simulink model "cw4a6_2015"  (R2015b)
settings: Solver=FixedStepAuto  SolverMode=SingleTasking  StartTime=0.0  StopTime=100  FixedStep=0.01  RelTol=1e-3
libraries: neural x31

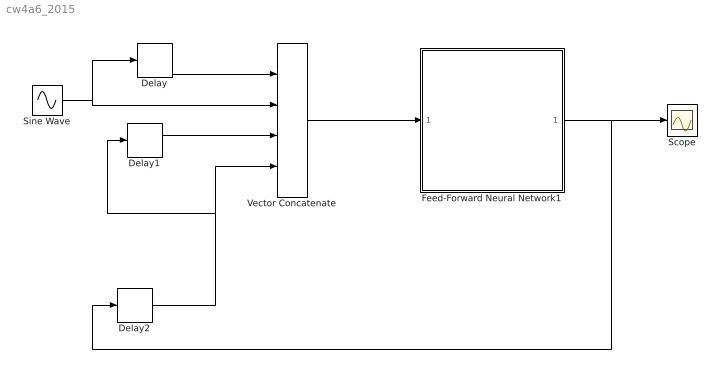
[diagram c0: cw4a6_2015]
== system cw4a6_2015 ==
  Delay : Delay  DelayLength=1  InitialCondition=0
  Delay1 : Delay  DelayLength=1  InitialCondition=0
  Delay2 : Delay  DelayLength=1  InitialCondition=0
  Feed-Forward Neural Network1 : Subsystem
  Scope : Scope
  Sine Wave : Sin  Amplitude=3  SampleTime=0
  Vector Concatenate : Concatenate  NumInputs=4
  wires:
  Vector Concatenate/1 -> Feed-Forward Neural Network1/1(Input)
  Sine Wave/1 -> Delay/1, Vector Concatenate/2
  Delay/1 -> Vector Concatenate/1
  Feed-Forward Neural Network1/1(Output) -> Scope/1, Delay2/1
  Delay1/1 -> Vector Concatenate/3
  Delay2/1 -> Delay1/1, Vector Concatenate/4

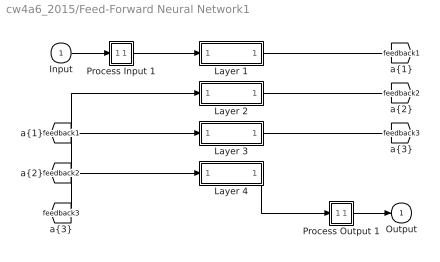
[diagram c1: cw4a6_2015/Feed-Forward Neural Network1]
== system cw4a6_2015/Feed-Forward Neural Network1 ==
  Input : Inport  PortDimensions=4  SampleTime=0.01
  Layer 1 : Subsystem
  Layer 2 : Subsystem
  Layer 3 : Subsystem
  Layer 4 : Subsystem
  Process Input 1 : Subsystem
  Process Output 1 : Subsystem
  Output : Outport  InitialOutput=0
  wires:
  Input/1 -> Process Input 1/1(x)
  Process Output 1/1(y) -> Output/1
  Process Input 1/1(p) -> Layer 1/1("p{1}")
  Layer 1/1("a{1}") -> [feedback1]
  [feedback1] -> Layer 2/1("a{1} ")
  Layer 2/1("a{2}") -> [feedback2]
  [feedback2] -> Layer 3/1("a{2} ")
  Layer 3/1("a{3}") -> [feedback3]
  [feedback3] -> Layer 4/1("a{3} ")
  Layer 4/1("a{4}") -> Process Output 1/1(a)

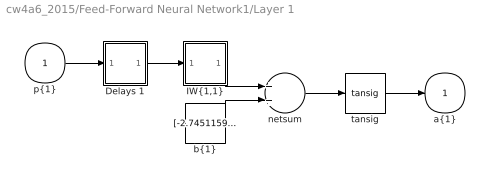
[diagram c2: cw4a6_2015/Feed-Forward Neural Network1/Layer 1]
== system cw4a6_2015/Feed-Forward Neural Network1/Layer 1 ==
  "p{1}" : Inport  PortDimensions=4  SampleTime=0.01
  Delays 1 : Subsystem
  "IW{1,1}" : Subsystem
  "b{1}" : Constant  Value=[-2.7451159693212377;-0.51927762787376885;1.1959405771862848;1.954048280311202]
  netsum : Sum  Inputs=2
  tansig : neural/Transfer Functions/tansig
  "a{1}" : Outport  InitialOutput=[0;0;0;0]
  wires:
  "p{1}"/1 -> Delays 1/1("p{1}")
  Delays 1/1("pd{1,1}") -> "IW{1,1}"/1("pd{1,1}")
  "IW{1,1}"/1("iz{1,1}") -> netsum/1
  "b{1}"/1 -> netsum/2
  netsum/1 -> tansig/1
  tansig/1 -> "a{1}"/1

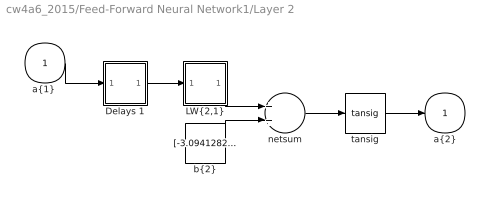
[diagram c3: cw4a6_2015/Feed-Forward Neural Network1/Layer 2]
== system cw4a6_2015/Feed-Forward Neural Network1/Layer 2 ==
  "a{1} " : Inport  PortDimensions=4  SampleTime=0.01
  Delays 1 : Subsystem
  "LW{2,1}" : Subsystem
  "b{2}" : Constant  Value=[-3.0941282887806971;2.5007190554093581;1.9491510266515135;-1.6091889436891094;1.4251518713600293;-1.2415776302483117;0.76744618770440332;-0.24724036630592988;0.4711224294363367;-0.70575018159961311;0.68364287193172868;-1.3894845729981458;1.1167616282660546;-2.0699518501358609;-2.3105194954019512;2.6036849767045065]
  netsum : Sum  Inputs=2
  tansig : neural/Transfer Functions/tansig
  "a{2}" : Outport  InitialOutput=[0;0;0;0;0;0;0;0;0;0;0;0;0;0;0;0]
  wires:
  "a{1} "/1 -> Delays 1/1("p{2}")
  Delays 1/1("pd{2,1}") -> "LW{2,1}"/1("ad{2,1}")
  "LW{2,1}"/1("lz{2,1}") -> netsum/1
  "b{2}"/1 -> netsum/2
  netsum/1 -> tansig/1
  tansig/1 -> "a{2}"/1

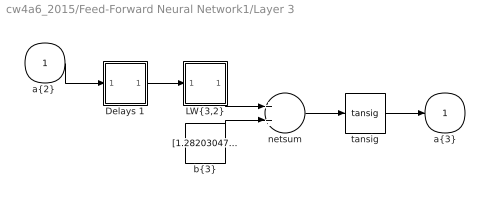
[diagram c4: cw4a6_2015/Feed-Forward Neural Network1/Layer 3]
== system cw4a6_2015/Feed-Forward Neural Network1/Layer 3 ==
  "a{2} " : Inport  PortDimensions=16  SampleTime=0.01
  Delays 1 : Subsystem
  "LW{3,2}" : Subsystem
  "b{3}" : Constant  Value=[1.2820304787533141;-0.73780855735148043;-0.35364559770692083;-1.5031025952607859]
  netsum : Sum  Inputs=2
  tansig : neural/Transfer Functions/tansig
  "a{3}" : Outport  InitialOutput=[0;0;0;0]
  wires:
  "a{2} "/1 -> Delays 1/1("p{3}")
  Delays 1/1("pd{3,2}") -> "LW{3,2}"/1("ad{3,2}")
  "LW{3,2}"/1("lz{3,2}") -> netsum/1
  "b{3}"/1 -> netsum/2
  netsum/1 -> tansig/1
  tansig/1 -> "a{3}"/1

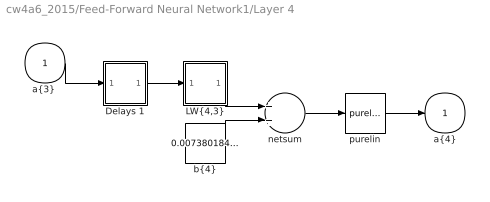
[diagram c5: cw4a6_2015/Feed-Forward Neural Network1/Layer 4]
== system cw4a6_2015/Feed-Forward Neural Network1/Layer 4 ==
  "a{3} " : Inport  PortDimensions=4  SampleTime=0.01
  Delays 1 : Subsystem
  "LW{4,3}" : Subsystem
  "b{4}" : Constant  Value=0.0073801844453347783
  netsum : Sum  Inputs=2
  purelin : neural/Transfer Functions/purelin
  "a{4}" : Outport  InitialOutput=0
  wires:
  "a{3} "/1 -> Delays 1/1("p{4}")
  Delays 1/1("pd{4,3}") -> "LW{4,3}"/1("ad{4,3}")
  "LW{4,3}"/1("lz{4,3}") -> netsum/1
  "b{4}"/1 -> netsum/2
  netsum/1 -> purelin/1
  purelin/1 -> "a{4}"/1

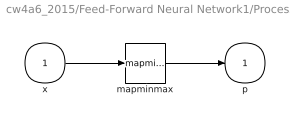
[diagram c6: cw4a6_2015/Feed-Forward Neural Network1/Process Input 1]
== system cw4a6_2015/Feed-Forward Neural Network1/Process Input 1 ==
  x : Inport  PortDimensions=4  SampleTime=0.01
  mapminmax : neural/Processing Functions/mapminmax  xmin=[-2.9999999573670899;-2.9999999573670899;-1.6037325965643041;-1.6037325965643041]  xmax=[2.9999999873508418;2.9999999873508418;1.5876018327536372;1.5876018327536372]  ymin=-1  ymax=1
  p : Outport  PortDimensions=4  SampleTime=0.01
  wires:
  x/1 -> mapminmax/1
  mapminmax/1 -> p/1

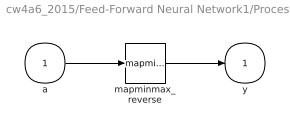
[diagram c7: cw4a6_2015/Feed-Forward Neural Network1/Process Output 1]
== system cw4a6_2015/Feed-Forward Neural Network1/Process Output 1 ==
  a : Inport  PortDimensions=1  SampleTime=0.01
  mapminmax_reverse : neural/Processing Functions/mapminmax_reverse  xmin=-1.6037325965643041  xmax=1.5876018327536372  ymin=-1  ymax=1
  y : Outport  PortDimensions=1  SampleTime=0.01
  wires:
  a/1 -> mapminmax_reverse/1
  mapminmax_reverse/1 -> y/1

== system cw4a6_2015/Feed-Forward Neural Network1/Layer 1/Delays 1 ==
  "p{1}" : Inport  PortDimensions=4  SampleTime=0.01
  mux : Mux  Inputs=1
  "pd{1,1}" : Outport
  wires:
  "p{1}"/1 -> mux/1
  mux/1 -> "pd{1,1}"/1

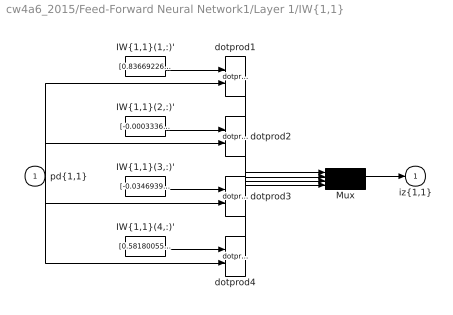
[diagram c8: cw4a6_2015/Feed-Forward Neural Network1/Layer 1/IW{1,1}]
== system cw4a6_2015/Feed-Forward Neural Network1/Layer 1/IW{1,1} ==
  "pd{1,1}" : Inport  PortDimensions=4  SampleTime=0.01
  "IW{1,1}(1,:)'" : Constant  Value=[0.83669226565768351;-0.74873759136295048;-0.96234576370289271;0.37325137038861117]
  "IW{1,1}(2,:)'" : Constant  Value=[-0.0003336744559937728;-0.00039010697089592478;-0.30642803603807789;0.60937703466284387]
  "IW{1,1}(3,:)'" : Constant  Value=[-0.034693924814063352;0.16844250588365894;0.76279626784045285;-0.17752775686451444]
  "IW{1,1}(4,:)'" : Constant  Value=[0.5818005537766594;0.90179528476757986;-0.22477921341837884;0.12222051479645338]
  Mux : Mux
  dotprod{1..4} (4 alike) : neural/Weight Functions/dotprod
  "iz{1,1}" : Outport
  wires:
  "IW{1,1}(1,:)'"/1 -> dotprod1/1
  "pd{1,1}"/1 -> dotprod1/2, dotprod2/2, dotprod3/2, dotprod4/2
  dotprod1/1 -> Mux/1
  "IW{1,1}(2,:)'"/1 -> dotprod2/1
  dotprod2/1 -> Mux/2
  "IW{1,1}(3,:)'"/1 -> dotprod3/1
  dotprod3/1 -> Mux/3
  "IW{1,1}(4,:)'"/1 -> dotprod4/1
  dotprod4/1 -> Mux/4
  Mux/1 -> "iz{1,1}"/1

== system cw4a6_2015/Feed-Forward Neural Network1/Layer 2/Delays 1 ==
  "p{2}" : Inport  PortDimensions=4  SampleTime=0.01
  mux : Mux  Inputs=1
  "pd{2,1}" : Outport
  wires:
  "p{2}"/1 -> mux/1
  mux/1 -> "pd{2,1}"/1

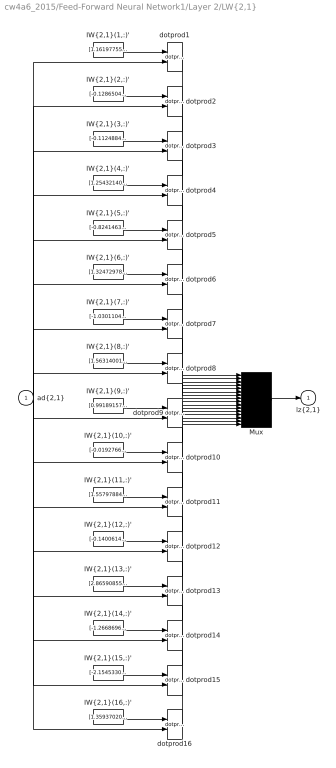
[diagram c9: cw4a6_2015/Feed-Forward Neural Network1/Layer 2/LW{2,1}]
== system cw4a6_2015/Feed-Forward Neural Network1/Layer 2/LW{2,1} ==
  "ad{2,1}" : Inport  PortDimensions=4  SampleTime=0.01
  "IW{2,1}(1,:)'" : Constant  Value=[1.1619775513977304;-2.2031284357403633;0.45459113386422795;-0.86857666926111776]
  "IW{2,1}(10,:)'" : Constant  Value=[-0.019276692855536848;0.54978083604503003;-1.3930468139942518;2.1350487871589929]
  "IW{2,1}(11,:)'" : Constant  Value=[1.5579788444873723;-1.5886105818001446;-1.0902860786850852;1.4211623229204338]
  "IW{2,1}(12,:)'" : Constant  Value=[-0.14006142548391878;-1.4133972790272766;-1.5916388419386516;1.5759542712752714]
  "IW{2,1}(13,:)'" : Constant  Value=[2.8659085537820359;0.60522502995712779;0.0058109977953483254;1.2254165100910313]
  "IW{2,1}(14,:)'" : Constant  Value=[-1.2668696691178363;2.0172300742823461;1.8445786770211106;0.26217247906200308]
  "IW{2,1}(15,:)'" : Constant  Value=[-2.1545330363134259;-0.64742657934957937;1.0991901026838413;-1.1935631889128151]
  "IW{2,1}(16,:)'" : Constant  Value=[1.3593702063748641;0.46413197701403974;2.3128596993208599;-0.12255806313010746]
  "IW{2,1}(2,:)'" : Constant  Value=[-0.12865042340396424;1.8582424739004237;1.2150803047094694;-1.2142721671715175]
  "IW{2,1}(3,:)'" : Constant  Value=[-0.11248842580797785;0.89804609193892571;1.8927709477903503;-1.8989976446848842]
  "IW{2,1}(4,:)'" : Constant  Value=[1.2543214069614295;-1.1815005524957249;-1.5671094633574423;1.5819257759203105]
  "IW{2,1}(5,:)'" : Constant  Value=[-0.82414639837216042;-1.9068075047638195;-1.8175012039809864;0.78505691762512242]
  "IW{2,1}(6,:)'" : Constant  Value=[1.3247297822434136;-1.4039801264342664;0.23930805038668623;-1.8575388549116805]
  "IW{2,1}(7,:)'" : Constant  Value=[-1.0301104085961448;-2.1013505254009393;-1.4127876628063598;0.9588134099123895]
  "IW{2,1}(8,:)'" : Constant  Value=[1.5631400167839289;-1.916152108882349;-0.011644069876120409;-0.24742781400878255]
  "IW{2,1}(9,:)'" : Constant  Value=[0.99189157553799678;-1.5265997169883485;2.2592796000731861;-0.088815072125645364]
  Mux : Mux  Inputs=16
  dotprod{1..16} (16 alike) : neural/Weight Functions/dotprod
  "lz{2,1}" : Outport
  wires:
  "IW{2,1}(1,:)'"/1 -> dotprod1/1
  "ad{2,1}"/1 -> dotprod1/2, dotprod2/2, dotprod3/2, dotprod4/2, dotprod5/2, dotprod6/2, dotprod7/2, dotprod8/2, dotprod9/2, dotprod10/2, dotprod11/2, dotprod12/2, dotprod13/2, dotprod14/2, dotprod15/2, dotprod16/2
  dotprod1/1 -> Mux/1
  "IW{2,1}(2,:)'"/1 -> dotprod2/1
  dotprod2/1 -> Mux/2
  "IW{2,1}(3,:)'"/1 -> dotprod3/1
  dotprod3/1 -> Mux/3
  "IW{2,1}(4,:)'"/1 -> dotprod4/1
  dotprod4/1 -> Mux/4
  "IW{2,1}(5,:)'"/1 -> dotprod5/1
  dotprod5/1 -> Mux/5
  "IW{2,1}(6,:)'"/1 -> dotprod6/1
  dotprod6/1 -> Mux/6
  "IW{2,1}(7,:)'"/1 -> dotprod7/1
  dotprod7/1 -> Mux/7
  "IW{2,1}(8,:)'"/1 -> dotprod8/1
  dotprod8/1 -> Mux/8
  "IW{2,1}(9,:)'"/1 -> dotprod9/1
  dotprod9/1 -> Mux/9
  "IW{2,1}(10,:)'"/1 -> dotprod10/1
  dotprod10/1 -> Mux/10
  "IW{2,1}(11,:)'"/1 -> dotprod11/1
  dotprod11/1 -> Mux/11
  "IW{2,1}(12,:)'"/1 -> dotprod12/1
  dotprod12/1 -> Mux/12
  "IW{2,1}(13,:)'"/1 -> dotprod13/1
  dotprod13/1 -> Mux/13
  "IW{2,1}(14,:)'"/1 -> dotprod14/1
  dotprod14/1 -> Mux/14
  "IW{2,1}(15,:)'"/1 -> dotprod15/1
  dotprod15/1 -> Mux/15
  "IW{2,1}(16,:)'"/1 -> dotprod16/1
  dotprod16/1 -> Mux/16
  Mux/1 -> "lz{2,1}"/1

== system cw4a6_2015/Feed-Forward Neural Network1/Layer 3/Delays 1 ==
  "p{3}" : Inport  PortDimensions=16  SampleTime=0.01
  mux : Mux  Inputs=1
  "pd{3,2}" : Outport
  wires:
  "p{3}"/1 -> mux/1
  mux/1 -> "pd{3,2}"/1

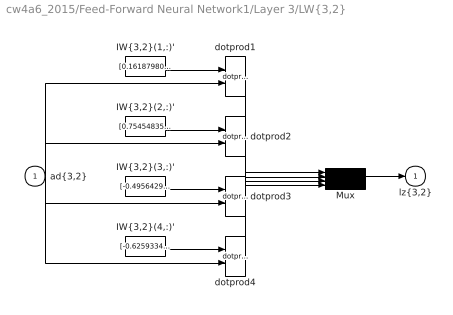
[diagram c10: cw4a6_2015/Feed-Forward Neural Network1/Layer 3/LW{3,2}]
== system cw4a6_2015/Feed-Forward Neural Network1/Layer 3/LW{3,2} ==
  "ad{3,2}" : Inport  PortDimensions=16  SampleTime=0.01
  "IW{3,2}(1,:)'" : Constant  Value=[0.16187980152970616;-0.012069549631443587;-0.33619237419074488;-0.11221275186314425;-0.84527343254795939;-0.13838173443262566;-0.86579761805405597;-0.54372197052752236;-0.5540698037394719;0.29642693101710327;-0.51600417022592104;0.12328800989395178;-0.023120032481970174;0.10739195901251349;-0.091127333814782302;0.3448023234057801]
  "IW{3,2}(2,:)'" : Constant  Value=[0.75454835221691474;0.15013552620515574;0.11472578766906887;0.42274443593459643;-0.39961601700928129;0.68875970158928868;-0.61849028246128845;-0.20169161472368685;0.75597763951241503;-0.28078016497474889;0.35272734174223885;0.15533241825389357;-0.54022006214681251;0.44824258664502548;0.20670522893995144;0.0021272597366931213]
  "IW{3,2}(3,:)'" : Constant  Value=[-0.49564299601633494;-0.59554041291666426;0.11518124790025119;0.4158342871985139;0.42913101457060854;0.057765199972912039;0.96450526133528924;0.74784337338286055;0.55940689624420914;0.061052507718161814;0.19601073852766301;0.1887571760997073;0.11904905216730757;0.0020121948030143583;0.54408499407374489;-0.75181015468307]
  "IW{3,2}(4,:)'" : Constant  Value=[-0.62593341733336327;-0.068162072264553578;0.70449927506796517;-0.57856612570268351;0.35167636963900833;0.3604973101877027;0.48372273273793348;-0.029178613812122785;0.11436187455567905;-0.19063994024956235;-0.020488469690563053;-0.012726413172482024;-0.97976764164592023;-0.98044237566603998;0.35726750753906772;0.24954643189041284]
  Mux : Mux
  dotprod{1..4} (4 alike) : neural/Weight Functions/dotprod
  "lz{3,2}" : Outport
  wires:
  "IW{3,2}(1,:)'"/1 -> dotprod1/1
  "ad{3,2}"/1 -> dotprod1/2, dotprod2/2, dotprod3/2, dotprod4/2
  dotprod1/1 -> Mux/1
  "IW{3,2}(2,:)'"/1 -> dotprod2/1
  dotprod2/1 -> Mux/2
  "IW{3,2}(3,:)'"/1 -> dotprod3/1
  dotprod3/1 -> Mux/3
  "IW{3,2}(4,:)'"/1 -> dotprod4/1
  dotprod4/1 -> Mux/4
  Mux/1 -> "lz{3,2}"/1

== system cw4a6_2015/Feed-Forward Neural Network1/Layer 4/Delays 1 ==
  "p{4}" : Inport  PortDimensions=4  SampleTime=0.01
  mux : Mux  Inputs=1
  "pd{4,3}" : Outport
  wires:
  "p{4}"/1 -> mux/1
  mux/1 -> "pd{4,3}"/1

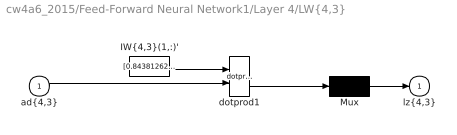
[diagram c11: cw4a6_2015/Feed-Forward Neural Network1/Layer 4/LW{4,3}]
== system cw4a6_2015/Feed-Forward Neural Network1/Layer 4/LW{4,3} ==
  "ad{4,3}" : Inport  PortDimensions=4  SampleTime=0.01
  "IW{4,3}(1,:)'" : Constant  Value=[0.84381262330633844;0.14088410255099024;-2.3372869652868911;-0.21203014435834328]
  Mux : Mux  Inputs=1
  dotprod1 : neural/Weight Functions/dotprod
  "lz{4,3}" : Outport
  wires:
  "IW{4,3}(1,:)'"/1 -> dotprod1/1
  "ad{4,3}"/1 -> dotprod1/2
  dotprod1/1 -> Mux/1
  Mux/1 -> "lz{4,3}"/1
